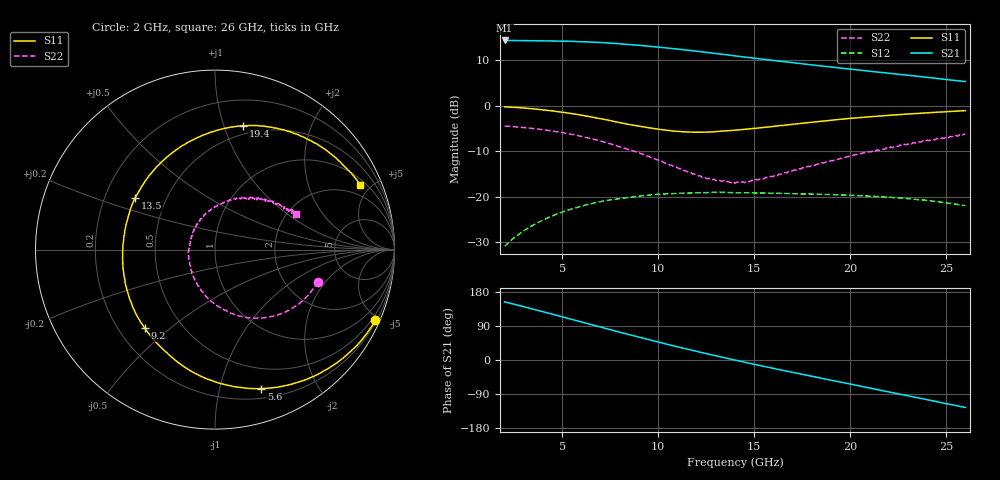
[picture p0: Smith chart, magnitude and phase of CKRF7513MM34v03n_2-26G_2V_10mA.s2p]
! CHUO DENSHI KOGYO Co.,Ltd.
! 22. July 2016
! CKRF7513MM34
! N-channel HJ-FET
! Vds = 2 V Id = 10 mA
# Hz S  MA  R 50
!	f	S11	S21	S12	S22
!	Hz	MAG	ANG	MAG	ANG	MAG	ANG	MAG	ANG
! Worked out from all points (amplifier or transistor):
!   241 points, 2 GHz to 26 GHz, reference 50 ohm
!   highest |S21| = 14.4 dB at 2 GHz (marker M1)
!   |S21| within 3 dB of that: start of sweep to 13.26 GHz
!   unconditionally stable (mu >= 1): 13.63 GHz to 20.39 GHz; 20.4321 GHz to 20.51526 GHz
!   at 6 GHz: K = 0.54, MSG = 18.1 dB, |S12| = -22.1 dB
!   at 14 GHz: K = 1.02, MAG = 14.2 dB, |S12| = -19.1 dB
!   at 26 GHz: K = 0.80, MSG = 13.7 dB, |S12| = -22.0 dB
!   lowest NFmin = 0.33 dB at 10 GHz
!   S11 on the Smith chart (normalised r, x): 2 GHz: 0.28, -4.72; 5.6 GHz: 0.29, -1.35; 9.2 GHz: 0.31, -0.41; 13.5 GHz: 0.33, +0.27; 19.4 GHz: 0.42, +1.17; 26 GHz: 1.31, +4.33
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2e9  0.9766 -23.8  5.252 153.6  0.0285 73.4  0.5999 -17.4
3e9  0.9459 -36.3  5.234 140.6  0.0421 65.4  0.5776 -26.3
4e9  0.9046 -49.2  5.211 127.4  0.05528 57.2  0.5458 -35.6
4.8e9  0.8635 -60.2  5.181 116.7  0.06537 50.4  0.5158 -43.3
5.6e9  0.8159 -71.6  5.129 105.9  0.07445 43.8  0.4817 -51.4
6e9  0.7903 -77.5  5.099 100.5  0.07874 40.5  0.4615 -55.6
6.7e9  0.7434 -88.5  5.024 91.0  0.08565 34.7  0.4251 -63.2
7.4e9  0.6948 -100.0  4.931 81.4  0.09151 28.9  0.3864 -71.2
8.1e9  0.6458 -112.0  4.803 72.0  0.09561 23.4  0.3476 -79.3
9.2e9  0.5877 -131.7  4.606 57.8  0.1026 15.6  0.2939 -92.6
1e10  0.553 -147.3  4.445 47.4  0.1057 9.8  0.254 -105.0
1.08e10  0.5284 -163.0  4.269 37.3  0.1082 4.3  0.2145 -117.9
1.17e10  0.5133 179.6  4.065 26.3  0.11 -1.4  0.185 -134.6
1.26e10  0.5148 162.8  3.862 15.6  0.111 -6.6  0.1582 -153.1
1.35e10  0.5308 147.0  3.664 5.1  0.1116 -12.4  0.1445 -177.6
1.4e10  0.5391 139.1  3.553 -0.5  0.1106 -15.0  0.1407 170.4
1.59e10  0.5914 113.2  3.181 -21.1  0.1094 -24.3  0.1671 129.2
1.8e10  0.6599 90.2  2.824 -42.9  0.1068 -33.8  0.2207 98.2
1.94e10  0.708 77.1  2.623 -57.3  0.1046 -40.3  0.2587 82.0
2.2e10  0.7858 55.2  2.289 -83.9  0.09869 -52.9  0.3375 56.3
2.41e10  0.8424 38.2  2.05 -105.8  0.09048 -63.8  0.4151 38.1
2.6e10  0.885 24.0  1.854 -125.3  0.0798 -74.0  0.4919 24.1
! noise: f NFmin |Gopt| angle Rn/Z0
1e+10  0.33  0.485  95.7  0.07
1.05e+10  0.35  0.471  104.3  0.06
1.1e+10  0.37  0.436  111.9  0.06
1.15e+10  0.39  0.405  123  0.05
1.2e+10  0.41  0.386  133.7  0.04
1.25e+10  0.43  0.36  144.2  0.04
1.3e+10  0.45  0.342  156.9  0.04
1.35e+10  0.48  0.339  169.1  0.03
1.4e+10  0.5  0.342  -178.8  0.03
1.5e+10  0.54  0.367  -156.6  0.04
